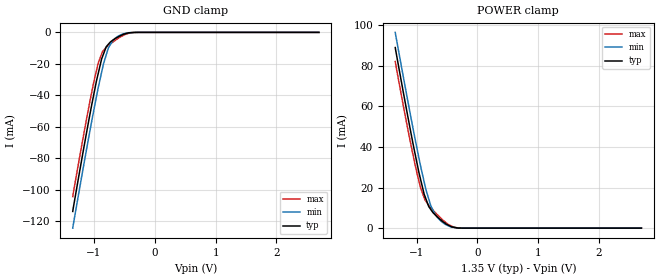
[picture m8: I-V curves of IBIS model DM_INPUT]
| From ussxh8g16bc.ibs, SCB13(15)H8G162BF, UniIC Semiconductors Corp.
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| MODEL DM_INPUT (DM Input Model with no ODT, 800-2133Mbps)
[Model]   DM_INPUT
Model_type   Input
Vinl = 545.000mV
Vinh = 805.000mV
|   typ   min   max
|C_comp   0.950pF   0.900pF   1.000pF
C_comp_power_clamp   0.4750pF   0.4500pF   0.5000pF
C_comp_gnd_clamp   0.4750pF   0.4500pF   0.5000pF
[Model Spec]
| Input threshold voltage corners
Vinl   0.5450V   0.5115V   0.5825V
Vinh   0.8050V   0.7715V   0.8425V
| Dynamic Overshoot Parameters from DDR3L Specification
|D_overshoot_ampl_h   0.40   NA   NA
|D_overshoot_ampl_l   0.40   NA   NA
|D_overshoot_area_h   0.11n   NA   NA
|D_overshoot_area_l   0.11n   NA   NA
[Receiver Thresholds]
Vth   =  0.675V
Vth_min  =  0.6615V
Vth_max  =  0.6885V
Vinh_ac  =  0.130V
Vinh_dc  =  0.090V
Vinl_ac  = -0.130V
Vinl_dc  = -0.090V
Tslew_ac =  5.000ns |Not specified, so set to high value
Threshold_sensitivity = 0.50
Reference_supply Power_clamp_ref
[Voltage Range]   1.3500V   1.2830V   1.4250V
[POWER Clamp Reference]   1.3500V   1.2830V   1.4250V
| Junction Temperature (Ambient temp is 40C typ, 85C min, 0C max)
[Temperature Range]   45.0   90.0   0.0
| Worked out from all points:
|   GND clamp passes 1 mA (typ) near -0.50 V on its own axis
|   POWER clamp passes 1 mA (typ) near -0.45 V on its own axis
[GND Clamp]
|   Voltage   I(typ)   I(min)   I(max)
-1.35V    -113.9mA   -124.6mA   -104.5mA
-1.205V   -81.48mA   -92.16mA   -72.46mA
-1.07V    -52.65mA   -63.14mA   -44.3mA
-1V       -38.7mA    -48.81mA   -30.85mA
-930mV    -25.95mA   -35.02mA   -19.4mA
-875mV    -16.88mA   -25.36mA   -13.69mA
-800mV    -9.222mA   -14.41mA   -9.487mA
-765mV    -7.604mA   -9.974mA   -8.359mA
-650mV    -3.918mA   -3.687mA   -5.017mA
-520mV    -1.303mA   -937.1uA   -1.955mA
-315mV    -19.67uA   -18.79uA   -28.64uA
2.7V      0A         0A         0A
[POWER Clamp]
|   Voltage   I(typ)   I(min)   I(max)
-1.35V    88.89mA    96.37mA    82.02mA
-1.205V   64.87mA    72.5mA     58.31mA
-1.07V    43.46mA    51mA       37.77mA
-930mV    23.58mA    30.09mA    19.57mA
-875mV    16.77mA    22.82mA    15.04mA
-800mV    10.68mA    14.43mA    11.22mA
-765mV    9.147mA    10.97mA    10.01mA
-690mV    6.433mA    6.617mA    7.571mA
-565mV    3.162mA    2.653mA    3.926mA
-395mV    485.8uA    358.5uA    537uA
-310mV    60.31uA    60.42uA    66.72uA
2.7V      0A         0A         0A
